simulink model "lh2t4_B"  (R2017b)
settings: Solver=ode45  StartTime=0.0  StopTime=10  RelTol=1e-3  EnableMultiTasking=on
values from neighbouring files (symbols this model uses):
  m0 = 1000    [lh2t4_DOC.m]
libraries: mat24129_lib x2

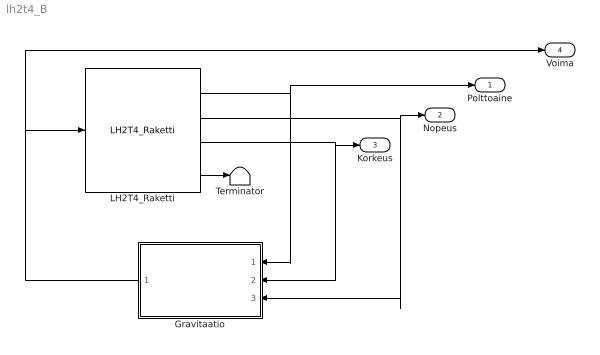
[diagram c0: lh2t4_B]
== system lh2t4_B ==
  Gravitaatio : Subsystem
  LH2T4_Raketti : mat24129_lib/LH2T4_Raketti
  Terminator : Terminator
  Polttoaine : Outport
  Nopeus : Outport  Port=2
  Korkeus : Outport  Port=3
  Voima : Outport  Port=4
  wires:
  LH2T4_Raketti/1 -> Polttoaine/1, Gravitaatio/1(Polttoaine)
  LH2T4_Raketti/2 -> Nopeus/1, Gravitaatio/3(Nopeus)
  LH2T4_Raketti/3 -> Korkeus/1, Gravitaatio/2(Korkeus)
  Gravitaatio/1(Voima) -> Voima/1, LH2T4_Raketti/1
  LH2T4_Raketti/4 -> Terminator/1

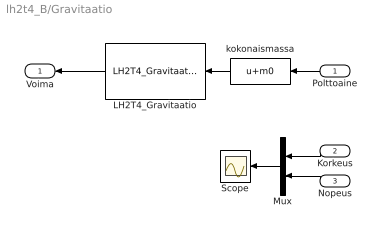
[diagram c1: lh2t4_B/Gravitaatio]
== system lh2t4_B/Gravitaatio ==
  Polttoaine : Inport
  Korkeus : Inport  Port=2
  Nopeus : Inport  Port=3
  LH2T4_Gravitaatio : mat24129_lib/LH2T4_Gravitaatio
  Mux : Mux  Inputs=2
  Scope : Scope
  kokonaismassa : Fcn  Expr=u+m0
  Voima : Outport
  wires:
  Mux/1 -> Scope/1
  Polttoaine/1 -> kokonaismassa/1
  Korkeus/1 -> Mux/1
  Nopeus/1 -> Mux/2
  kokonaismassa/1 -> LH2T4_Gravitaatio/1
  LH2T4_Gravitaatio/1 -> Voima/1
